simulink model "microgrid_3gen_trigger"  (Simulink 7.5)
settings: Solver=ode23tb  StartTime=0.0  StopTime=20  FixedStep=0.001  RelTol=1e-4
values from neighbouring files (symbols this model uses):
  A = [A_ele, -A_ele, 0    [run_microgrid_3gen_trigger.m]
  B = [2*A_ele,-A_ele,A_ele    [run_microgrid_3gen_trigger.m]
  Ereq1 = 1    [run_microgrid_3gen_trigger.m]
  Ereq2 = 1    [run_microgrid_3gen_trigger.m]
  Ereq3 = 1    [run_microgrid_3gen_trigger.m]
  flag_trigger = 0    [run_microgrid_3gen_trigger.m]
  gen_b = [0.1,1.8,0.5]    [run_microgrid_3gen_trigger.m]
  gen_c = [0.1,0.1,0.1]    [run_microgrid_3gen_trigger.m]
  Ki = 750*160    (= 120000)    [run_microgrid_3gen_trigger.m]
  Kilim = 30    [run_microgrid_3gen_trigger.m]
  Kp = 750*0.001    (= 0.75)    [run_microgrid_3gen_trigger.m]
  Kplim = 0    [run_microgrid_3gen_trigger.m]
  Lgen = 0.00188    [run_microgrid_3gen_trigger.m]
  Lline12 = Lline    (= 1.0345071301e-05)    [run_microgrid_3gen_trigger.m]
  Lline23 = Lline    (= 1.0345071301e-05)    [run_microgrid_3gen_trigger.m]
  Lline31 = Lline    (= 1.0345071301e-05)    [run_microgrid_3gen_trigger.m]
  Lload1 = 0.001/w0    (= 2.65258238486e-06)    [run_microgrid_3gen_trigger.m]
  Lload2 = 0.001/w0    (= 2.65258238486e-06)    [run_microgrid_3gen_trigger.m]
  Lload3 = 0.001/w0    (= 2.65258238486e-06)    [run_microgrid_3gen_trigger.m]
  mP = pi    (= 3.14159265359)    [run_microgrid_3gen_trigger.m]
  mQ = 0.05    [run_microgrid_3gen_trigger.m]
  P_lim_d = [-.4,-.4,-.4]    [run_microgrid_3gen_trigger.m]
  P_lim_u = [.4,.4,.4]    [run_microgrid_3gen_trigger.m]
  Pgen_lim_d = [0.0,0.0,0.0]    [run_microgrid_3gen_trigger.m]
  Pgen_lim_u = [1.0,1.0,1.0]    [run_microgrid_3gen_trigger.m]
  Pmax = 1.0    (= 1)    [run_microgrid_3gen_trigger.m]
  Pmin = 0.0    (= 0)    [run_microgrid_3gen_trigger.m]
  Preq1 = 0.4    [run_microgrid_3gen_trigger.m]    (also in odyssian_4a_plot.m = Preq.signals(1).values; Power_Dispatcher.m = 1)
  Preq2 = 0.8    [run_microgrid_3gen_trigger.m]    (also in odyssian_4a_plot.m = Preq.signals(2).values; Power_Dispatcher.m = 1)
  Preq3 = 0.6    [run_microgrid_3gen_trigger.m]    (also in odyssian_4a_plot.m = Preq.signals(3).values; Power_Dispatcher.m = 1)
  Rline12 = Rline    (= 0)    [run_microgrid_3gen_trigger.m]
  Rline23 = Rline    (= 0)    [run_microgrid_3gen_trigger.m]
  Rline31 = Rline    (= 0)    [run_microgrid_3gen_trigger.m]
  Rload1 = 3    [run_microgrid_3gen_trigger.m]
  Rload2 = 4    [run_microgrid_3gen_trigger.m]
  Rload3 = 6    [run_microgrid_3gen_trigger.m]
  Sbase = 15000    [run_microgrid_3gen_trigger.m]
  t_trigger_start = 3    [run_microgrid_3gen_trigger.m]
  tau_Preq = 0.03    [run_microgrid_3gen_trigger.m]
  tauf = 0.03    [run_microgrid_3gen_trigger.m]
  Vbase = 208/sqrt(3)    [run_microgrid_3gen_trigger.m]
  w0 = 2.0*pi*60    (= 376.991118431)    [run_microgrid_3gen_trigger.m]
  w_d_gen = [w_gen,w_gen,w_gen]    [run_microgrid_3gen_trigger.m]
  w_d_link = [w_line;w_line;w_line]    [run_microgrid_3gen_trigger.m]
  w_u_gen = [w_gen,w_gen,w_gen]    [run_microgrid_3gen_trigger.m]
  w_u_link = [w_line;w_line;w_line]    [run_microgrid_3gen_trigger.m]
libraries: powerlib x73, powerlib_extras x3
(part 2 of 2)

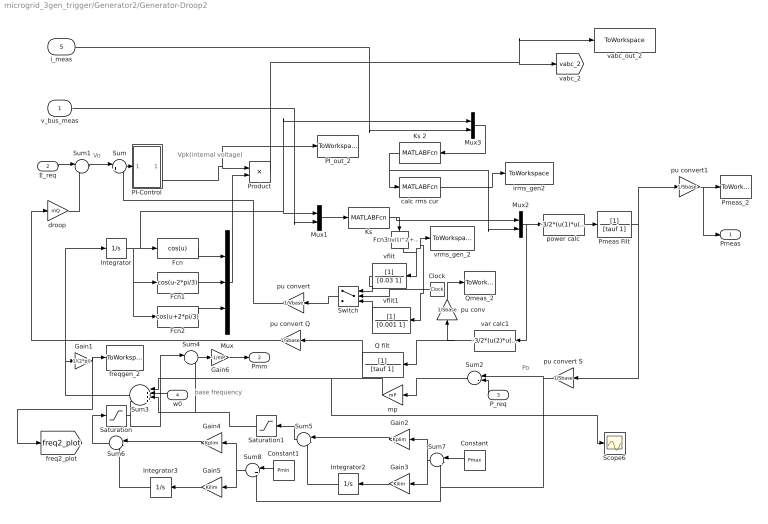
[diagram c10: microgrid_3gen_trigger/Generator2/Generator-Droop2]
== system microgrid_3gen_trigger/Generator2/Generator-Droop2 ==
  note: Vpk(internal voltage)
  note: Vo
  note: Po
  note: base frequency
  v_bus_meas : Inport
  E_req : Inport  Port=2
  P_req : Inport  Port=3
  w0 : Inport  Port=4
  i_meas : Inport  Port=5
  Clock : Clock
  Constant : Constant  Value=Pmax  OutDataType=sfix(16)  OutScaling=2^0
  Constant1 : Constant  Value=Pmin  OutDataType=sfix(16)  OutScaling=2^0
  Fcn : Fcn  Expr=cos(u)
  Fcn1 : Fcn  Expr=cos(u-2*pi/3)
  Fcn2 : Fcn  Expr=cos(u+2*pi/3)
  Fcn3 : Fcn  Expr=sqrt(u(1)^2 + u(2)^2)/sqrt(2)
  Gain1 : Gain  Gain=1/(2*pi)  ParameterDataType=sfix(16)  ParameterScaling=2^0  OutDataType=sfix(16)  OutScaling=2^0
  Gain2 : Gain  Gain=Kplim  ParameterDataType=sfix(16)  ParameterScaling=2^0  OutDataType=sfix(16)  OutScaling=2^0
  Gain3 : Gain  Gain=Kilim  ParameterDataType=sfix(16)  ParameterScaling=2^0  OutDataType=sfix(16)  OutScaling=2^0
  Gain4 : Gain  Gain=Kplim  ParameterDataType=sfix(16)  ParameterScaling=2^0  OutDataType=sfix(16)  OutScaling=2^0
  Gain5 : Gain  Gain=Kilim  ParameterDataType=sfix(16)  ParameterScaling=2^0  OutDataType=sfix(16)  OutScaling=2^0
  Gain6 : Gain  Gain=-1/mP  ParameterDataType=sfix(16)  ParameterScaling=2^0  OutDataType=sfix(16)  OutScaling=2^0
  Integrator : Integrator
  Integrator2 : Integrator  UpperSaturationLimit=0  LowerSaturationLimit=-2*pi
  Integrator3 : Integrator  UpperSaturationLimit=2*pi  LowerSaturationLimit=0
  Ks : MATLABFcn  MATLABFcn=Ks_
  Ks 2 : MATLABFcn  MATLABFcn=Ks_
  Mux : Mux  Inputs=3
  Mux1 : Mux  Inputs=2
  Mux2 : Mux  Inputs=2
  Mux3 : Mux  Inputs=2
  PI-Control : Subsystem
  PI_out_2 : ToWorkspace  VariableName=PI_out_2  SampleTime=-1  SaveFormat=Array
  Pmeas Filt : TransferFcn  Denominator=[tauf 1]
  Pmeas_2 : ToWorkspace  VariableName=Pmeas_2  SampleTime=-1  SaveFormat=Array
  Product : Product  OutDataType=sfix(16)  OutScaling=2^0
  Q filt : TransferFcn  Denominator=[tauf 1]
  Qmeas_2 : ToWorkspace  VariableName=Qmeas_2  SampleTime=-1  SaveFormat=Array
  Saturation : Saturate  UpperLimit=2*pi  LowerLimit=0  OutDataType=fixdt(1, 16)  OutScaling=2^0
  Saturation1 : Saturate  UpperLimit=0  LowerLimit=-2*pi  OutDataType=fixdt(1, 16)  OutScaling=2^0
  Scope6 : Scope
  Sum : Sum  Inputs=|+-  OutDataType=sfix(16)  OutScaling=2^0
  Sum{1,4..6} (4 alike) : Sum  Inputs=|++  OutDataType=sfix(16)  OutScaling=2^0
  Sum2 : Sum  Inputs=|-+  OutDataType=sfix(16)  OutScaling=2^0
  Sum3 : Sum  Inputs=|++++  OutDataType=sfix(16)  OutScaling=2^0
  Sum7 : Sum  Inputs=|+-  OutDataType=sfix(16)  OutScaling=2^0
  Sum8 : Sum  Inputs=|+-  OutDataType=sfix(16)  OutScaling=2^0
  Switch : Switch  Criteria=u2 > Threshold  Threshold=2  OutDataType=fixdt(1, 16)  OutScaling=2^0
  calc rms cur : MATLABFcn  MATLABFcn=RMS_
  "droop " : Gain  Gain=mQ  ParameterDataType=sfix(16)  ParameterScaling=2^0  OutDataType=sfix(16)  OutScaling=2^0
  freqgen_2 : ToWorkspace  VariableName=freqgen_2  SampleTime=-1  SaveFormat=Array
  irms_gen2 : ToWorkspace  VariableName=irms_gen_2  SampleTime=-1  SaveFormat=Array
  mp : Gain  Gain=mP  ParameterDataType=sfix(16)  ParameterScaling=2^0  OutDataType=sfix(16)  OutScaling=2^0
  power calc : Fcn  Expr=-3/2*(u(1)*u(4) + u(2)*u(5) + 2*u(3)*u(6))
  pu conv : Gain  Gain=1/Sbase  ParameterDataType=sfix(16)  ParameterScaling=2^0  OutDataType=sfix(16)  OutScaling=2^0
  pu convert : Gain  Gain=1/Vbase  ParameterDataType=sfix(16)  ParameterScaling=2^0  OutDataType=sfix(16)  OutScaling=2^0
  pu convert Q : Gain  Gain=1/Sbase  ParameterDataType=sfix(16)  ParameterScaling=2^0  OutDataType=sfix(16)  OutScaling=2^0
  pu convert S : Gain  Gain=1/Sbase  ParameterDataType=sfix(16)  ParameterScaling=2^0  OutDataType=sfix(16)  OutScaling=2^0
  pu convert1 : Gain  Gain=1/Sbase  ParameterDataType=sfix(16)  ParameterScaling=2^0  OutDataType=sfix(16)  OutScaling=2^0
  vabc_out_2 : ToWorkspace  VariableName=vabc_out_2  SampleTime=-1  SaveFormat=Array
  var calc1 : Fcn  Expr=-3/2*(u(2)*u(4) - u(1)*u(5))
  vflit : TransferFcn  Denominator=[0.03 1]
  vflit1 : TransferFcn  Denominator=[0.001 1]
  vrms_gen_2 : ToWorkspace  VariableName=vrms_gen_2  SampleTime=-1  SaveFormat=Array
  Pmeas : Outport  OutDataType=fixdt(1, 16)  OutScaling=2^0
  Pmm : Outport  Port=2  OutDataType=fixdt(1, 16)  OutScaling=2^0
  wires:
  Integrator/1 -> Fcn1/1, Fcn2/1, Fcn/1, Mux1/1, Mux3/1
  Fcn/1 -> Mux/1
  Fcn1/1 -> Mux/2
  Fcn2/1 -> Mux/3
  Mux/1 -> Product/2
  Sum1/1 -> Sum/1
  pu convert/1 -> Sum/2
  "droop "/1 -> Sum1/2
  pu convert S/1 -> Sum2/1, Sum7/2, Sum8/2
  Sum2/1 -> mp/1
  mp/1 -> Sum3/1, Scope6/1
  Sum3/1 -> Integrator/1, Gain1/1
  pu convert Q/1 -> "droop "/1
  Q filt/1 -> pu convert Q/1
  E_req/1 -> Sum1/1
  P_req/1 -> Sum2/2
  w0/1 -> Sum3/2
  Gain3/1 -> Integrator2/1
  Integrator2/1 -> Sum5/2
  Gain2/1 -> Sum5/1
  Gain5/1 -> Integrator3/1
  Integrator3/1 -> Sum6/2
  Gain4/1 -> Sum6/1
  Sum7/1 -> Gain2/1, Gain3/1
  Sum8/1 -> Gain5/1, Gain4/1
  Constant/1 -> Sum7/1
  Constant1/1 -> Sum8/1
  Sum/1 -> PI-Control/1(In1)
  calc rms cur/1 -> irms_gen2/1
  Mux3/1 -> Ks 2/1
  var calc1/1 -> Q filt/1, pu conv/1
  Ks 2/1 -> Mux2/2, calc rms cur/1
  Mux2/1 -> power calc/1, var calc1/1
  Mux1/1 -> Ks/1
  Fcn3/1 -> vflit/1, vrms_gen_2/1, vflit1/1
  Gain1/1 -> freqgen_2/1, [freq2_plot]
  Ks/1 -> Mux2/1, Fcn3/1
  v_bus_meas/1 -> Mux1/2
  pu convert1/1 -> Pmeas_2/1, Pmeas/1
  pu conv/1 -> Qmeas_2/1
  i_meas/1 -> Mux3/2
  Product/1 -> [vabc_2], vabc_out_2/1
  Sum6/1 -> Saturation/1
  Saturation/1 -> Sum3/4, Sum4/1
  Sum5/1 -> Saturation1/1
  Saturation1/1 -> Sum3/3, Sum4/2
  Sum4/1 -> Gain6/1
  Gain6/1 -> Pmm/1
  power calc/1 -> Pmeas Filt/1
  Pmeas Filt/1 -> pu convert S/1, pu convert1/1
  PI-Control/1(Out1) -> Product/1, PI_out_2/1
  vflit/1 -> Switch/1
  Switch/1 -> pu convert/1
  vflit1/1 -> Switch/3
  Clock/1 -> Switch/2

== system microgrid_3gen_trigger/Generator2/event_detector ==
  phi : Inport
  z : Inport  Port=2
  Demux : Demux  Outputs=2
  Mux2 : Mux  Inputs=2
  S-Function : S-Function  FunctionName=trigger_block  EnableBusSupport=off
  phi_hat : Outport
  tsamp : Outport  Port=2
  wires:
  Mux2/1 -> S-Function/1
  z/1 -> Mux2/2
  phi/1 -> Mux2/1
  Demux/2 -> tsamp/1
  Demux/1 -> phi_hat/1
  S-Function/1 -> Demux/1

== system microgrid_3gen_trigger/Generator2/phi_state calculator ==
  P_meas : Inport
  Mux1 : Mux  Inputs=3
  Mux2 : Mux  Inputs=5
  Pgen_lim_d : Constant  Value=Pgen_lim_d(2)  OutDataType=sfix(16)  OutScaling=2^0
  Pgen_lim_u : Constant  Value=Pgen_lim_u(2)  OutDataType=sfix(16)  OutScaling=2^0
  Sum1 : Sum  Inputs=|++  OutDataType=sfix(16)  OutScaling=2^0
  gen_b : Constant  Value=gen_b(2)  OutDataType=sfix(16)  OutScaling=2^0
  gen_c : Constant  Value=gen_c(2)  OutDataType=sfix(16)  OutScaling=2^0
  phi_state : Fcn  Expr=u(2)+2*u(3)*u(1)
  phi_state1 : MATLABFcn  MATLABFcn=phi_state
  w_d_gen : Constant  Value=w_d_gen(2)  OutDataType=sfix(16)  OutScaling=2^0
  w_u_gen : Constant  Value=w_u_gen(2)  OutDataType=sfix(16)  OutScaling=2^0
  phi : Outport  OutDataType=fixdt(1, 16)  OutScaling=2^0
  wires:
  Mux1/1 -> phi_state/1
  gen_c/1 -> Mux1/3
  P_meas/1 -> Mux1/1, Mux2/1
  gen_b/1 -> Mux1/2
  Mux2/1 -> phi_state1/1
  w_u_gen/1 -> Mux2/2
  Pgen_lim_u/1 -> Mux2/3
  w_d_gen/1 -> Mux2/4
  Pgen_lim_d/1 -> Mux2/5
  phi_state1/1 -> Sum1/2
  phi_state/1 -> Sum1/1
  Sum1/1 -> phi/1

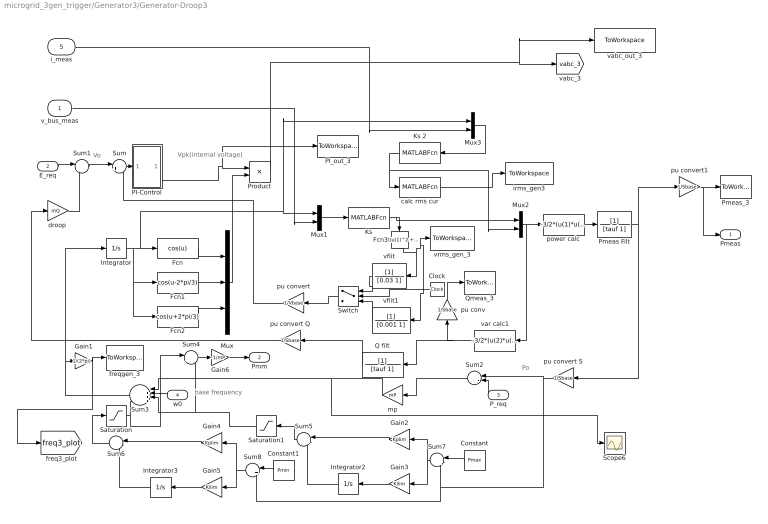
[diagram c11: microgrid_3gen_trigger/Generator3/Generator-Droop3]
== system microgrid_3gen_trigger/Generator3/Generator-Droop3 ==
  note: Vpk(internal voltage)
  note: Vo
  note: Po
  note: base frequency
  v_bus_meas : Inport
  E_req : Inport  Port=2
  P_req : Inport  Port=3
  w0 : Inport  Port=4
  i_meas : Inport  Port=5
  Clock : Clock
  Constant : Constant  Value=Pmax  OutDataType=sfix(16)  OutScaling=2^0
  Constant1 : Constant  Value=Pmin  OutDataType=sfix(16)  OutScaling=2^0
  Fcn : Fcn  Expr=cos(u)
  Fcn1 : Fcn  Expr=cos(u-2*pi/3)
  Fcn2 : Fcn  Expr=cos(u+2*pi/3)
  Fcn3 : Fcn  Expr=sqrt(u(1)^2 + u(2)^2)/sqrt(2)
  Gain1 : Gain  Gain=1/(2*pi)  ParameterDataType=sfix(16)  ParameterScaling=2^0  OutDataType=sfix(16)  OutScaling=2^0
  Gain2 : Gain  Gain=Kplim  ParameterDataType=sfix(16)  ParameterScaling=2^0  OutDataType=sfix(16)  OutScaling=2^0
  Gain3 : Gain  Gain=Kilim  ParameterDataType=sfix(16)  ParameterScaling=2^0  OutDataType=sfix(16)  OutScaling=2^0
  Gain4 : Gain  Gain=Kplim  ParameterDataType=sfix(16)  ParameterScaling=2^0  OutDataType=sfix(16)  OutScaling=2^0
  Gain5 : Gain  Gain=Kilim  ParameterDataType=sfix(16)  ParameterScaling=2^0  OutDataType=sfix(16)  OutScaling=2^0
  Gain6 : Gain  Gain=-1/mP  ParameterDataType=sfix(16)  ParameterScaling=2^0  OutDataType=sfix(16)  OutScaling=2^0
  Integrator : Integrator
  Integrator2 : Integrator  UpperSaturationLimit=0  LowerSaturationLimit=-2*pi
  Integrator3 : Integrator  UpperSaturationLimit=2*pi  LowerSaturationLimit=0
  Ks : MATLABFcn  MATLABFcn=Ks_
  Ks 2 : MATLABFcn  MATLABFcn=Ks_
  Mux : Mux  Inputs=3
  Mux1 : Mux  Inputs=2
  Mux2 : Mux  Inputs=2
  Mux3 : Mux  Inputs=2
  PI-Control : Subsystem
  PI_out_3 : ToWorkspace  VariableName=PI_out_3  SampleTime=-1  SaveFormat=Array
  Pmeas Filt : TransferFcn  Denominator=[tauf 1]
  Pmeas_3 : ToWorkspace  VariableName=Pmeas_3  SampleTime=-1  SaveFormat=Array
  Product : Product  OutDataType=sfix(16)  OutScaling=2^0
  Q filt : TransferFcn  Denominator=[tauf 1]
  Qmeas_3 : ToWorkspace  VariableName=Qmeas_3  SampleTime=-1  SaveFormat=Array
  Saturation : Saturate  UpperLimit=2*pi  LowerLimit=0  OutDataType=fixdt(1, 16)  OutScaling=2^0
  Saturation1 : Saturate  UpperLimit=0  LowerLimit=-2*pi  OutDataType=fixdt(1, 16)  OutScaling=2^0
  Scope6 : Scope
  Sum : Sum  Inputs=|+-  OutDataType=sfix(16)  OutScaling=2^0
  Sum{1,4..6} (4 alike) : Sum  Inputs=|++  OutDataType=sfix(16)  OutScaling=2^0
  Sum2 : Sum  Inputs=|-+  OutDataType=sfix(16)  OutScaling=2^0
  Sum3 : Sum  Inputs=|++++  OutDataType=sfix(16)  OutScaling=2^0
  Sum7 : Sum  Inputs=|+-  OutDataType=sfix(16)  OutScaling=2^0
  Sum8 : Sum  Inputs=|+-  OutDataType=sfix(16)  OutScaling=2^0
  Switch : Switch  Criteria=u2 > Threshold  Threshold=2  OutDataType=fixdt(1, 16)  OutScaling=2^0
  calc rms cur : MATLABFcn  MATLABFcn=RMS_
  "droop " : Gain  Gain=mQ  ParameterDataType=sfix(16)  ParameterScaling=2^0  OutDataType=sfix(16)  OutScaling=2^0
  freqgen_3 : ToWorkspace  VariableName=freqgen_3  SampleTime=-1  SaveFormat=Array
  irms_gen3 : ToWorkspace  VariableName=irms_gen_3  SampleTime=-1  SaveFormat=Array
  mp : Gain  Gain=mP  ParameterDataType=sfix(16)  ParameterScaling=2^0  OutDataType=sfix(16)  OutScaling=2^0
  power calc : Fcn  Expr=-3/2*(u(1)*u(4) + u(2)*u(5) + 2*u(3)*u(6))
  pu conv : Gain  Gain=1/Sbase  ParameterDataType=sfix(16)  ParameterScaling=2^0  OutDataType=sfix(16)  OutScaling=2^0
  pu convert : Gain  Gain=1/Vbase  ParameterDataType=sfix(16)  ParameterScaling=2^0  OutDataType=sfix(16)  OutScaling=2^0
  pu convert Q : Gain  Gain=1/Sbase  ParameterDataType=sfix(16)  ParameterScaling=2^0  OutDataType=sfix(16)  OutScaling=2^0
  pu convert S : Gain  Gain=1/Sbase  ParameterDataType=sfix(16)  ParameterScaling=2^0  OutDataType=sfix(16)  OutScaling=2^0
  pu convert1 : Gain  Gain=1/Sbase  ParameterDataType=sfix(16)  ParameterScaling=2^0  OutDataType=sfix(16)  OutScaling=2^0
  vabc_out_3 : ToWorkspace  VariableName=vabc_out_3  SampleTime=-1  SaveFormat=Array
  var calc1 : Fcn  Expr=-3/2*(u(2)*u(4) - u(1)*u(5))
  vflit : TransferFcn  Denominator=[0.03 1]
  vflit1 : TransferFcn  Denominator=[0.001 1]
  vrms_gen_3 : ToWorkspace  VariableName=vrms_gen_3  SampleTime=-1  SaveFormat=Array
  Pmeas : Outport  OutDataType=fixdt(1, 16)  OutScaling=2^0
  Pmm : Outport  Port=2  OutDataType=fixdt(1, 16)  OutScaling=2^0
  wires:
  Integrator/1 -> Fcn1/1, Fcn2/1, Fcn/1, Mux1/1, Mux3/1
  Fcn/1 -> Mux/1
  Fcn1/1 -> Mux/2
  Fcn2/1 -> Mux/3
  Mux/1 -> Product/2
  Sum1/1 -> Sum/1
  pu convert/1 -> Sum/2
  "droop "/1 -> Sum1/2
  pu convert S/1 -> Sum2/1, Sum7/2, Sum8/2
  Sum2/1 -> mp/1
  mp/1 -> Sum3/1, Scope6/1
  Sum3/1 -> Integrator/1, Gain1/1
  pu convert Q/1 -> "droop "/1
  Q filt/1 -> pu convert Q/1
  E_req/1 -> Sum1/1
  P_req/1 -> Sum2/2
  w0/1 -> Sum3/2
  Gain3/1 -> Integrator2/1
  Integrator2/1 -> Sum5/2
  Gain2/1 -> Sum5/1
  Gain5/1 -> Integrator3/1
  Integrator3/1 -> Sum6/2
  Gain4/1 -> Sum6/1
  Sum7/1 -> Gain2/1, Gain3/1
  Sum8/1 -> Gain5/1, Gain4/1
  Constant/1 -> Sum7/1
  Constant1/1 -> Sum8/1
  Sum/1 -> PI-Control/1(In1)
  calc rms cur/1 -> irms_gen3/1
  Mux3/1 -> Ks 2/1
  var calc1/1 -> Q filt/1, pu conv/1
  Ks 2/1 -> Mux2/2, calc rms cur/1
  Mux2/1 -> power calc/1, var calc1/1
  Mux1/1 -> Ks/1
  Fcn3/1 -> vflit/1, vrms_gen_3/1, vflit1/1
  Gain1/1 -> freqgen_3/1, [freq3_plot]
  Ks/1 -> Mux2/1, Fcn3/1
  v_bus_meas/1 -> Mux1/2
  pu convert1/1 -> Pmeas_3/1, Pmeas/1
  pu conv/1 -> Qmeas_3/1
  i_meas/1 -> Mux3/2
  Product/1 -> [vabc_3], vabc_out_3/1
  Sum6/1 -> Saturation/1
  Saturation/1 -> Sum3/4, Sum4/1
  Sum5/1 -> Saturation1/1
  Saturation1/1 -> Sum3/3, Sum4/2
  Sum4/1 -> Gain6/1
  Gain6/1 -> Pmm/1
  power calc/1 -> Pmeas Filt/1
  Pmeas Filt/1 -> pu convert S/1, pu convert1/1
  PI-Control/1(Out1) -> Product/1, PI_out_3/1
  vflit/1 -> Switch/1
  Switch/1 -> pu convert/1
  vflit1/1 -> Switch/3
  Clock/1 -> Switch/2

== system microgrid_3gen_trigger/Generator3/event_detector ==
  phi : Inport
  z : Inport  Port=2
  Demux : Demux  Outputs=2
  Mux2 : Mux  Inputs=2
  S-Function : S-Function  FunctionName=trigger_block  EnableBusSupport=off
  phi_hat : Outport
  tsamp : Outport  Port=2
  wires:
  Mux2/1 -> S-Function/1
  z/1 -> Mux2/2
  phi/1 -> Mux2/1
  Demux/2 -> tsamp/1
  Demux/1 -> phi_hat/1
  S-Function/1 -> Demux/1

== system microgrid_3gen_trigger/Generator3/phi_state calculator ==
  P_meas : Inport
  Mux1 : Mux  Inputs=3
  Mux2 : Mux  Inputs=5
  Pgen_lim_d : Constant  Value=Pgen_lim_d(3)  OutDataType=sfix(16)  OutScaling=2^0
  Pgen_lim_u : Constant  Value=Pgen_lim_u(3)  OutDataType=sfix(16)  OutScaling=2^0
  Sum1 : Sum  Inputs=|++  OutDataType=sfix(16)  OutScaling=2^0
  gen_b : Constant  Value=gen_b(3)  OutDataType=sfix(16)  OutScaling=2^0
  gen_c : Constant  Value=gen_c(3)  OutDataType=sfix(16)  OutScaling=2^0
  phi_state : Fcn  Expr=u(2)+2*u(3)*u(1)
  phi_state1 : MATLABFcn  MATLABFcn=phi_state
  w_d_gen : Constant  Value=w_d_gen(3)  OutDataType=sfix(16)  OutScaling=2^0
  w_u_gen : Constant  Value=w_u_gen(3)  OutDataType=sfix(16)  OutScaling=2^0
  phi : Outport  OutDataType=fixdt(1, 16)  OutScaling=2^0
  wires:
  Mux1/1 -> phi_state/1
  gen_c/1 -> Mux1/3
  P_meas/1 -> Mux1/1, Mux2/1
  gen_b/1 -> Mux1/2
  Mux2/1 -> phi_state1/1
  w_u_gen/1 -> Mux2/2
  Pgen_lim_u/1 -> Mux2/3
  w_d_gen/1 -> Mux2/4
  Pgen_lim_d/1 -> Mux2/5
  phi_state1/1 -> Sum1/2
  phi_state/1 -> Sum1/1
  Sum1/1 -> phi/1

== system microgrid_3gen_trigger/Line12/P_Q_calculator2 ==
  v : Inport
  i : Inport  Port=2
  Mux2 : Mux  Inputs=2
  P calculator : Fcn  Expr=((u(2)-u(3))*u(6) - (u(1)-u(2))*u(4))/Sbase
  Q calculator : Fcn  Expr="-(  (u(2)-u(3))*(2*u(4)+u(5)) +(u(3)-u(1))*(2*u(5)+u(4))  )/Sbase/sqrt(3)"
  P : Outport  OutDataType=fixdt(1, 16)  OutScaling=2^0
  Q : Outport  Port=2  OutDataType=fixdt(1, 16)  OutScaling=2^0
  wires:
  v/1 -> Mux2/1
  i/1 -> Mux2/2
  Mux2/1 -> P calculator/1, Q calculator/1
  P calculator/1 -> P/1
  Q calculator/1 -> Q/1

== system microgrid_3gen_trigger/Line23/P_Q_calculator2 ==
  v : Inport
  i : Inport  Port=2
  Mux2 : Mux  Inputs=2
  P calculator : Fcn  Expr=((u(2)-u(3))*u(6) - (u(1)-u(2))*u(4))/Sbase
  Q calculator : Fcn  Expr="-(  (u(2)-u(3))*(2*u(4)+u(5)) +(u(3)-u(1))*(2*u(5)+u(4))  )/Sbase/sqrt(3)"
  P : Outport  OutDataType=fixdt(1, 16)  OutScaling=2^0
  Q : Outport  Port=2  OutDataType=fixdt(1, 16)  OutScaling=2^0
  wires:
  v/1 -> Mux2/1
  i/1 -> Mux2/2
  Mux2/1 -> P calculator/1, Q calculator/1
  P calculator/1 -> P/1
  Q calculator/1 -> Q/1

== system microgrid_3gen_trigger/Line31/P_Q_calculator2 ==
  v : Inport
  i : Inport  Port=2
  Mux2 : Mux  Inputs=2
  P calculator : Fcn  Expr=((u(2)-u(3))*u(6) - (u(1)-u(2))*u(4))/Sbase
  Q calculator : Fcn  Expr="-(  (u(2)-u(3))*(2*u(4)+u(5)) +(u(3)-u(1))*(2*u(5)+u(4))  )/Sbase/sqrt(3)"
  P : Outport  OutDataType=fixdt(1, 16)  OutScaling=2^0
  Q : Outport  Port=2  OutDataType=fixdt(1, 16)  OutScaling=2^0
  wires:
  v/1 -> Mux2/1
  i/1 -> Mux2/2
  Mux2/1 -> P calculator/1, Q calculator/1
  P calculator/1 -> P/1
  Q calculator/1 -> Q/1

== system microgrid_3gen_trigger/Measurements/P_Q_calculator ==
  v : Inport
  i : Inport  Port=2
  Mux2 : Mux  Inputs=2
  P calculator : Fcn  Expr=((u(2)-u(3))*u(6) - (u(1)-u(2))*u(4))/Sbase
  Q calculator : Fcn  Expr="-(  (u(2)-u(3))*(2*u(4)+u(5)) +(u(3)-u(1))*(2*u(5)+u(4))  )/Sbase/sqrt(3)"
  P : Outport  OutDataType=fixdt(1, 16)  OutScaling=2^0
  Q : Outport  Port=2  OutDataType=fixdt(1, 16)  OutScaling=2^0
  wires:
  v/1 -> Mux2/1
  i/1 -> Mux2/2
  Mux2/1 -> P calculator/1, Q calculator/1
  P calculator/1 -> P/1
  Q calculator/1 -> Q/1

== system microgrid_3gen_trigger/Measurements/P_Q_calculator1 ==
  v : Inport
  i : Inport  Port=2
  Mux2 : Mux  Inputs=2
  P calculator : Fcn  Expr=((u(2)-u(3))*u(6) - (u(1)-u(2))*u(4))/Sbase
  Q calculator : Fcn  Expr="-(  (u(2)-u(3))*(2*u(4)+u(5)) +(u(3)-u(1))*(2*u(5)+u(4))  )/Sbase/sqrt(3)"
  P : Outport  OutDataType=fixdt(1, 16)  OutScaling=2^0
  Q : Outport  Port=2  OutDataType=fixdt(1, 16)  OutScaling=2^0
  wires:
  v/1 -> Mux2/1
  i/1 -> Mux2/2
  Mux2/1 -> P calculator/1, Q calculator/1
  P calculator/1 -> P/1
  Q calculator/1 -> Q/1

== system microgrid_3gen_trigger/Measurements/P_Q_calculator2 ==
  v : Inport
  i : Inport  Port=2
  Mux2 : Mux  Inputs=2
  P calculator : Fcn  Expr=((u(2)-u(3))*u(6) - (u(1)-u(2))*u(4))/Sbase
  Q calculator : Fcn  Expr="-(  (u(2)-u(3))*(2*u(4)+u(5)) +(u(3)-u(1))*(2*u(5)+u(4))  )/Sbase/sqrt(3)"
  P : Outport  OutDataType=fixdt(1, 16)  OutScaling=2^0
  Q : Outport  Port=2  OutDataType=fixdt(1, 16)  OutScaling=2^0
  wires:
  v/1 -> Mux2/1
  i/1 -> Mux2/2
  Mux2/1 -> P calculator/1, Q calculator/1
  P calculator/1 -> P/1
  Q calculator/1 -> Q/1

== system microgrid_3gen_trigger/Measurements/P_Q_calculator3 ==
  v : Inport
  i : Inport  Port=2
  Mux2 : Mux  Inputs=2
  P calculator : Fcn  Expr=((u(2)-u(3))*u(6) - (u(1)-u(2))*u(4))/Sbase
  Q calculator : Fcn  Expr="-(  (u(2)-u(3))*(2*u(4)+u(5)) +(u(3)-u(1))*(2*u(5)+u(4))  )/Sbase/sqrt(3)"
  P : Outport  OutDataType=fixdt(1, 16)  OutScaling=2^0
  Q : Outport  Port=2  OutDataType=fixdt(1, 16)  OutScaling=2^0
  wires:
  v/1 -> Mux2/1
  i/1 -> Mux2/2
  Mux2/1 -> P calculator/1, Q calculator/1
  P calculator/1 -> P/1
  Q calculator/1 -> Q/1

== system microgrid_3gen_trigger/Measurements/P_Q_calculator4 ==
  v : Inport
  i : Inport  Port=2
  Mux2 : Mux  Inputs=2
  P calculator : Fcn  Expr=((u(2)-u(3))*u(6) - (u(1)-u(2))*u(4))/Sbase
  Q calculator : Fcn  Expr="-(  (u(2)-u(3))*(2*u(4)+u(5)) +(u(3)-u(1))*(2*u(5)+u(4))  )/Sbase/sqrt(3)"
  P : Outport  OutDataType=fixdt(1, 16)  OutScaling=2^0
  Q : Outport  Port=2  OutDataType=fixdt(1, 16)  OutScaling=2^0
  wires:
  v/1 -> Mux2/1
  i/1 -> Mux2/2
  Mux2/1 -> P calculator/1, Q calculator/1
  P calculator/1 -> P/1
  Q calculator/1 -> Q/1

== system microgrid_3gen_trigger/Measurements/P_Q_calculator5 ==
  v : Inport
  i : Inport  Port=2
  Mux2 : Mux  Inputs=2
  P calculator : Fcn  Expr=((u(2)-u(3))*u(6) - (u(1)-u(2))*u(4))/Sbase
  Q calculator : Fcn  Expr="-(  (u(2)-u(3))*(2*u(4)+u(5)) +(u(3)-u(1))*(2*u(5)+u(4))  )/Sbase/sqrt(3)"
  P : Outport  OutDataType=fixdt(1, 16)  OutScaling=2^0
  Q : Outport  Port=2  OutDataType=fixdt(1, 16)  OutScaling=2^0
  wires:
  v/1 -> Mux2/1
  i/1 -> Mux2/2
  Mux2/1 -> P calculator/1, Q calculator/1
  P calculator/1 -> P/1
  Q calculator/1 -> Q/1

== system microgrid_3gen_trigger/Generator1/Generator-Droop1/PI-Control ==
  In1 : Inport
  Gain : Gain  Gain=Kp  ParameterDataType=sfix(16)  ParameterScaling=2^0  OutDataType=sfix(16)  OutScaling=2^0
  Gain1 : Gain  Gain=Ki  ParameterDataType=sfix(16)  ParameterScaling=2^0  OutDataType=sfix(16)  OutScaling=2^0
  Integrator1 : Integrator
  Sum4 : Sum  Inputs=|++  OutDataType=sfix(16)  OutScaling=2^0
  Out1 : Outport
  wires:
  Gain1/1 -> Integrator1/1
  In1/1 -> Gain/1, Gain1/1
  Integrator1/1 -> Sum4/2
  Gain/1 -> Sum4/1
  Sum4/1 -> Out1/1

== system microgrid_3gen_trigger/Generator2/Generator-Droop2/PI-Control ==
  In1 : Inport
  Gain : Gain  Gain=Kp  ParameterDataType=sfix(16)  ParameterScaling=2^0  OutDataType=sfix(16)  OutScaling=2^0
  Gain1 : Gain  Gain=Ki  ParameterDataType=sfix(16)  ParameterScaling=2^0  OutDataType=sfix(16)  OutScaling=2^0
  Integrator1 : Integrator
  Sum4 : Sum  Inputs=|++  OutDataType=sfix(16)  OutScaling=2^0
  Out1 : Outport
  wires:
  Gain1/1 -> Integrator1/1
  In1/1 -> Gain/1, Gain1/1
  Integrator1/1 -> Sum4/2
  Gain/1 -> Sum4/1
  Sum4/1 -> Out1/1

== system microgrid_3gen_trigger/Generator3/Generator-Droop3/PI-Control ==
  In1 : Inport
  Gain : Gain  Gain=Kp  ParameterDataType=sfix(16)  ParameterScaling=2^0  OutDataType=sfix(16)  OutScaling=2^0
  Gain1 : Gain  Gain=Ki  ParameterDataType=sfix(16)  ParameterScaling=2^0  OutDataType=sfix(16)  OutScaling=2^0
  Integrator1 : Integrator
  Sum4 : Sum  Inputs=|++  OutDataType=sfix(16)  OutScaling=2^0
  Out1 : Outport
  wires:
  Gain1/1 -> Integrator1/1
  In1/1 -> Gain/1, Gain1/1
  Integrator1/1 -> Sum4/2
  Gain/1 -> Sum4/1
  Sum4/1 -> Out1/1
